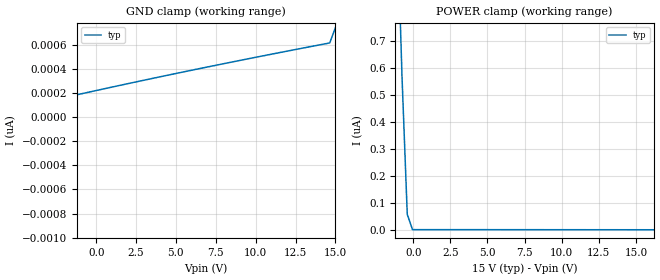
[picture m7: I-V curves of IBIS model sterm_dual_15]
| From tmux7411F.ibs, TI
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| sterm_dual_15
[Model]   sterm_dual_15
Model_type   Terminator
|   typ   min   max
C_comp   4.014581e-12   NA   NA
[Voltage Range]   15   NA   NA
[Temperature Range]   27   NA   NA
[Power Clamp Reference]   15   NA   NA
[GND Clamp Reference]   0   NA   NA
[GND Clamp]
|   Voltage   I(typ)   I(min)   I(max)
-20V      -17.87uA   NA         NA
-15.05V   -2.349nA   NA         NA
-14.7V    -176.4pA   NA         NA
-9.394V   -52.78pA   NA         NA
4.04V     335.3pA    NA         NA
14.65V    615.2pA    NA         NA
15V       740.9pA    NA         NA
[POWER Clamp]
|   Voltage   I(typ)   I(min)   I(max)
-5V       8.864uA    NA         NA
-1.111V   1.206uA    NA         NA
-757.6mV  567.4nA    NA         NA
-404mV    57.27nA    NA         NA
-50.5mV   754.1pA    NA         NA
30V       -622.9pA   NA         NA
